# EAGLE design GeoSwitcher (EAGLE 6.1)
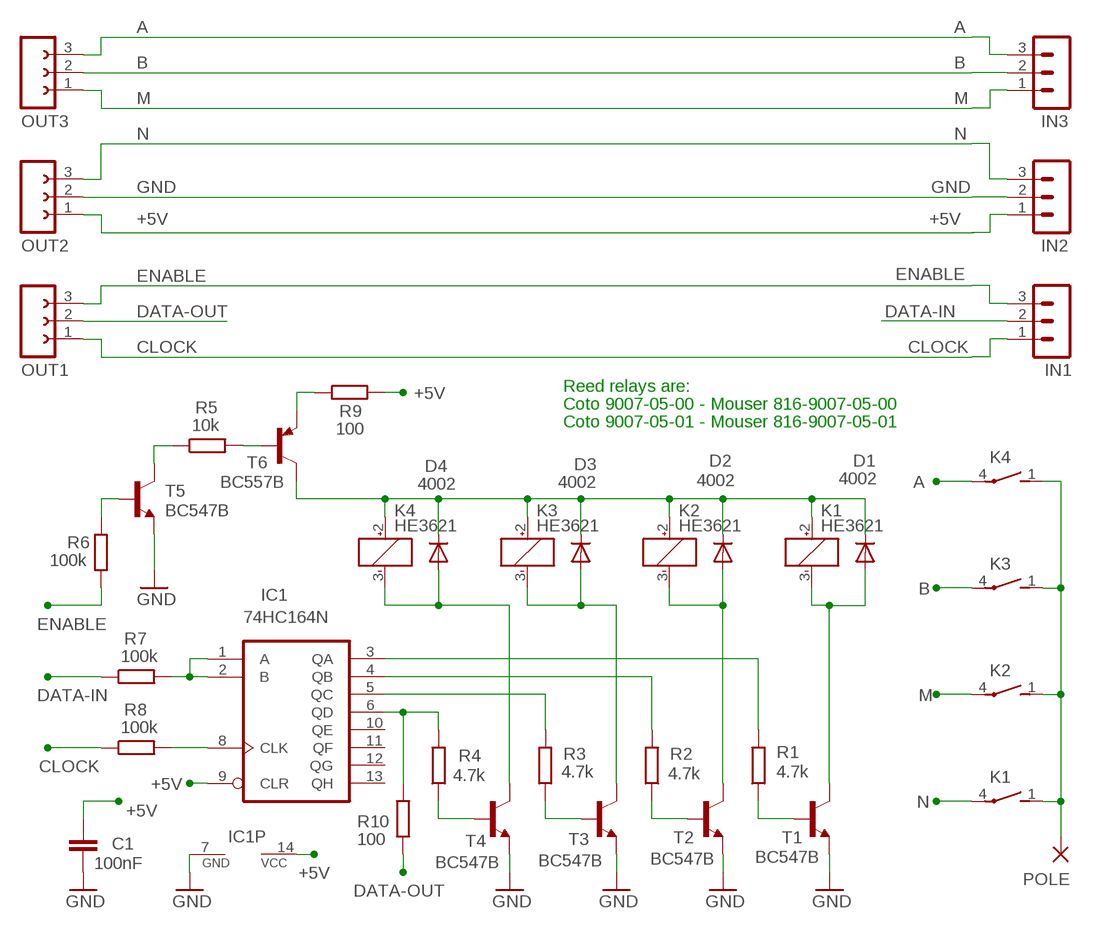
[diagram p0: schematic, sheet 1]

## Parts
C1  100nF  C-EU025-024X044  [C025-024X044]
D1  4002  DIODE-DO34-7  [DO34-7]
D2  4002  DIODE-DO34-7  [DO34-7]
D3  4002  DIODE-DO34-7  [DO34-7]
D4  4002  DIODE-DO34-7  [DO34-7]
IC1  74HC164N  [DIL14]
IN1  MA03-1N  [MA03-1]
IN2  MA03-1N  [MA03-1]
IN3  MA03-1N  [MA03-1]
K1  HE3621  [HE3621]
K2  HE3621  [HE3621]
K3  HE3621  [HE3621]
K4  HE3621  [HE3621]
OUT1  FE03-1"  [FE03-1]
OUT2  FE03-1"  [FE03-1]
OUT3  FE03-1"  [FE03-1]
POLE  WIREPAD2,54/0,8  [2,54/0,8]
R1  4.7k  R-EU_0204/7  [0204/7]
R2  4.7k  R-EU_0204/7  [0204/7]
R3  4.7k  R-EU_0204/7  [0204/7]
R4  4.7k  R-EU_0204/7  [0204/7]
R5  10k  R-EU_0204/7  [0204/7]
R6  100k  R-EU_0207/10  [0207/10]
R7  100k  R-EU_0207/12  [0207/12]
R8  100k  R-EU_0204/7  [0204/7]
R9  100  R-EU_0204/7  [0204/7]
R10  100  R-EU_0207/12  [0207/12]
T1  BC547B  -NPN-TO92-CBE  [TO92-CBE]
T2  BC547B  -NPN-TO92-CBE  [TO92-CBE]
T3  BC547B  -NPN-TO92-CBE  [TO92-CBE]
T4  BC547B  -NPN-TO92-CBE  [TO92-CBE]
T5  BC547B  -NPN-TO92-CBE  [TO92-CBE]
T6  BC557B  -PNP-TO92-CBE  [TO92-CBE]

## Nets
+5V: C1.1 IC1.9(CLR) IC1.14(VCC) IN2.1 OUT2.1 R9.2
A: IN3.3 K4.4(2:P) OUT3.3
B: IN3.2 K3.4(2:P) OUT3.2
CLOCK: IN1.1 OUT1.1 R8.1
DATA-IN: IN1.2 R7.1
DATA-OUT: OUT1.2 R10.1
ENABLE: IN1.3 OUT1.3 R6.2
GND: C1.2 IC1.7(GND) IN2.2 OUT2.2 T1.E T2.E T3.E T4.E T5.E
M: IN3.1 K2.4(2:P) OUT3.1
N: IN2.3 K1.4(2:P) OUT2.3
N$1: R4.1 T4.B
N$2: K1.1(2:S) K2.1(2:S) K3.1(2:S) K4.1(2:S) POLE.1(P)
N$3: D1.C D2.C D3.C D4.C K1.2(1:+) K2.2(1:+) K3.2(1:+) K4.2(1:+) T6.C
N$4: R3.1 T3.B
N$5: IC1.5(QC) R3.2
N$6: R2.1 T2.B
N$7: IC1.4(QB) R2.2
N$8: R1.1 T1.B
N$9: IC1.3(QA) R1.2
N$10: D4.A K4.3(1:-) T4.C
N$11: D3.A K3.3(1:-) T3.C
N$12: D2.A K2.3(1:-) T2.C
N$13: D1.A K1.3(1:-) T1.C
N$14: R5.1 T5.C
N$15: R5.2 T6.B
N$16: R6.1 T5.B
N$17: IC1.1(A) IC1.2(B) R7.2
N$18: IC1.8(CLK) R8.2
N$20: R9.1 T6.E
N$24: IC1.6(QD) R4.2 R10.2
Unconnected: IC1.10(QE) IC1.11(QF) IC1.12(QG) IC1.13(QH)

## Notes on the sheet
- Reed relays are:
- Coto 9007-05-00 - Mouser 816-9007-05-00
- Coto 9007-05-01 - Mouser 816-9007-05-01

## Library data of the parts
C1 = 00-LIVIO:C-EU: CAPACITOR, European symbol
D1-D4 = 00-LIVIO:DIODE-: DIODE
IC1 = 74xx-eu:74*164: 8-bit parallel out SHIFT REGISTER
IN1-IN3 = 03-con-lstb-M:MA03-1: PIN HEADER
K1-K4 = relay:HE3621: RELAY reed, 1 x norm. open, grid 5.08 mm, Hamlin
OUT1-OUT3 = 02-con-lsta-F:FE03-1: FEMALE HEADER
POLE = 00-LIVIO:WIREPAD: Wire PAD connect wire on PCB
R1-R10 = 00-LIVIO:R-EU_: RESISTOR, European symbol
T1-T5 = 00-LIVIO:*-NPN-: NPN Transistror
T6 = 00-LIVIO:*-PNP-: PNP Transistror

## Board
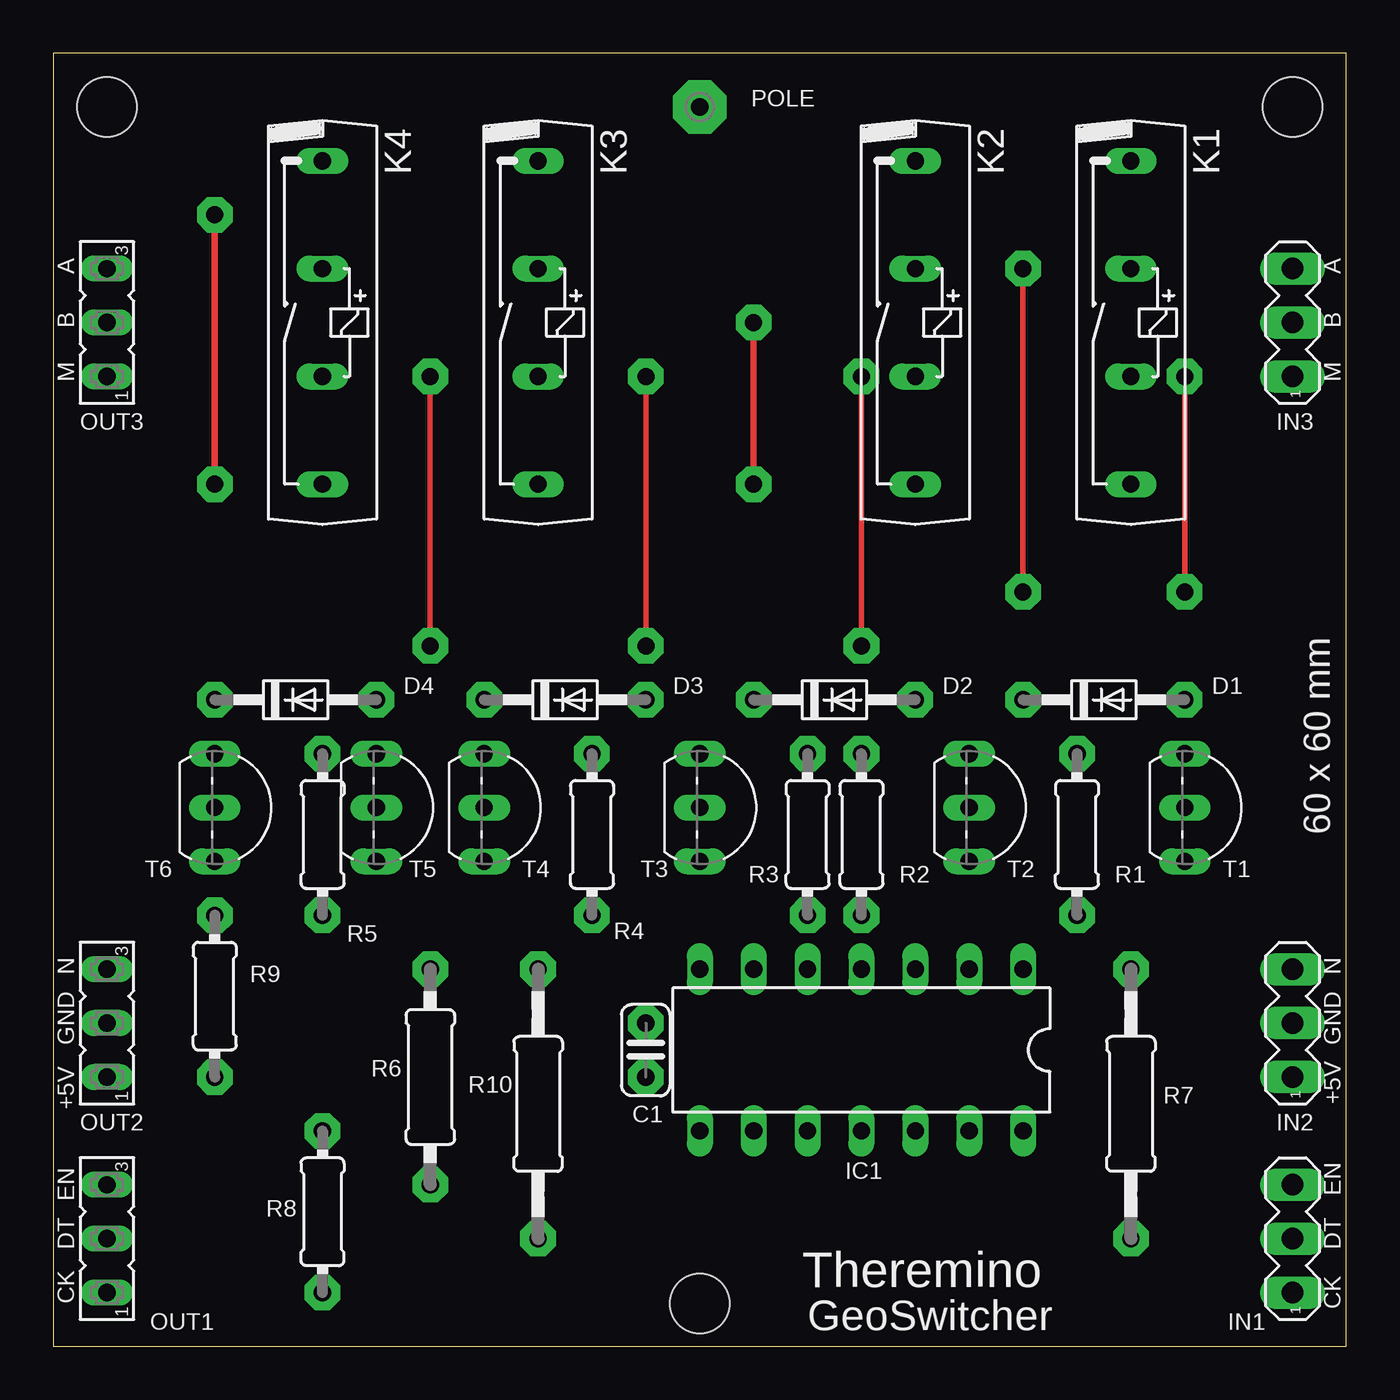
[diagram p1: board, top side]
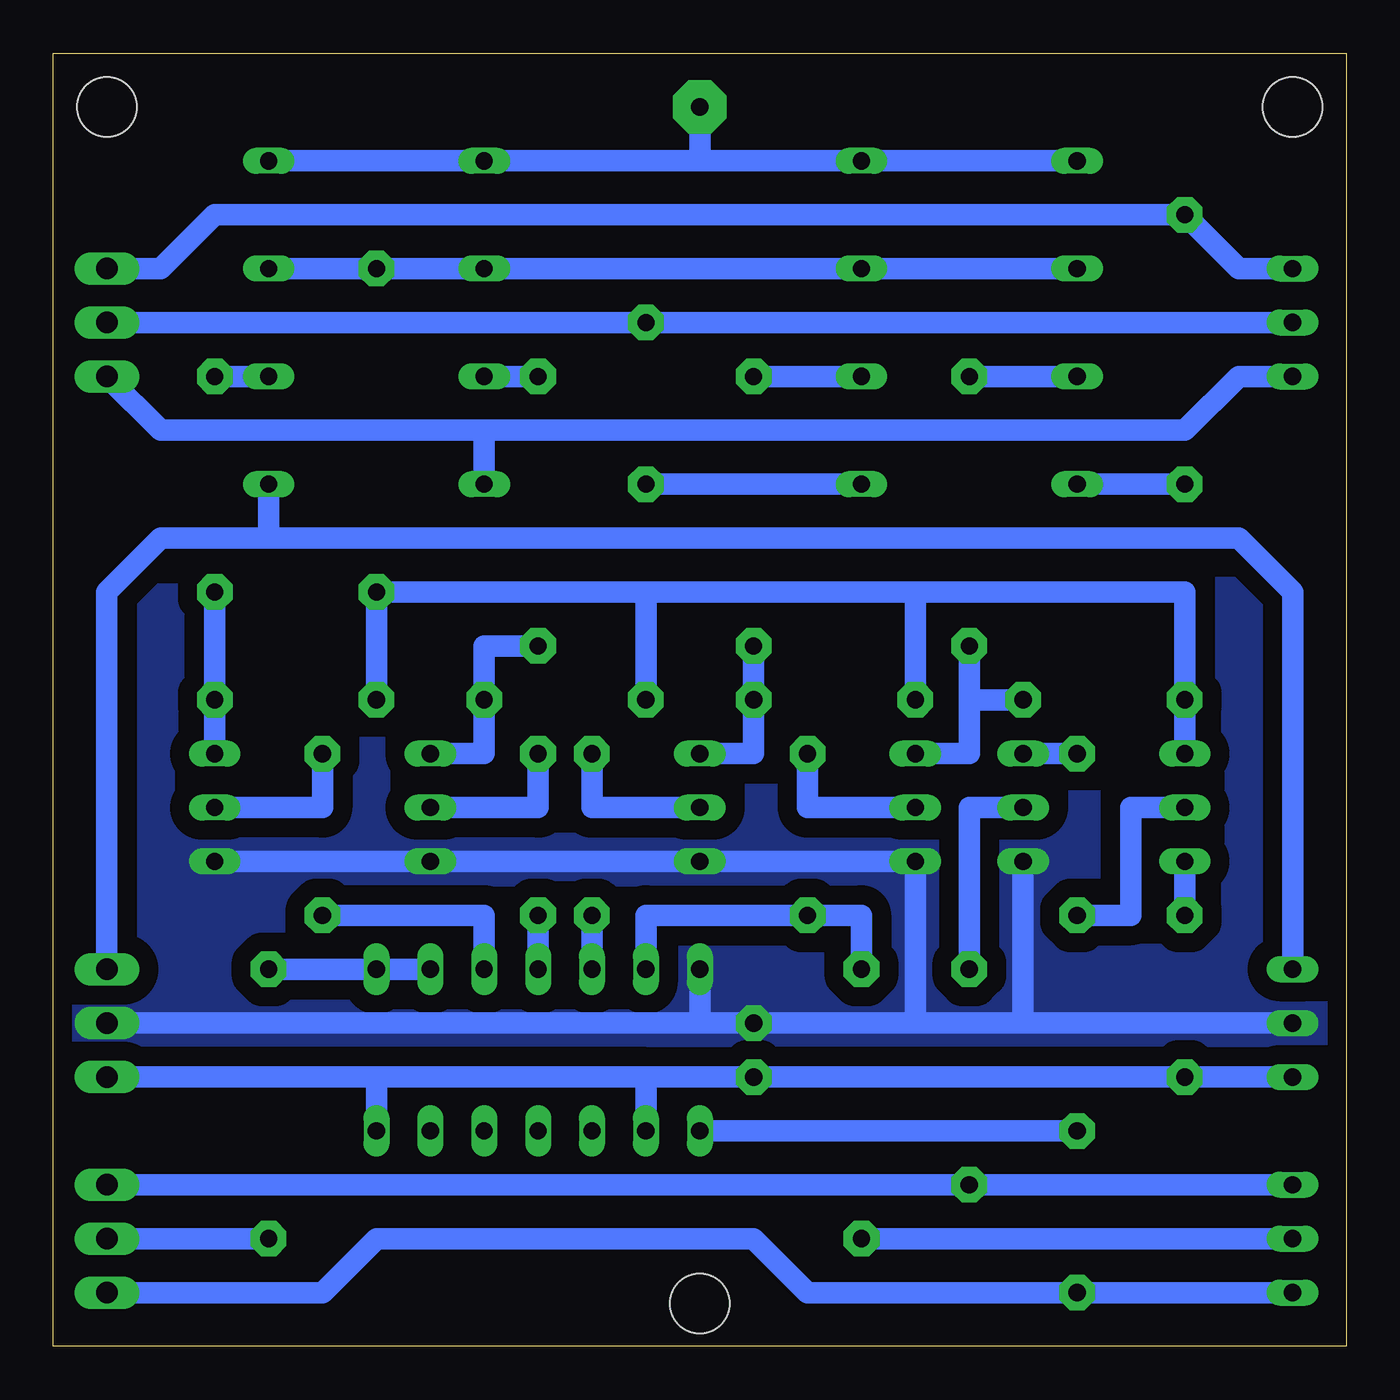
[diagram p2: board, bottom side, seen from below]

Size 60.96 x 60.96 mm. Coordinates in mm from the lower left corner, seen from the top.
Outline: 60.96,60.96 0,60.96 0,0 60.96,0 60.96,60.96
Copper layers (1*16): Top 0.035mm / dielectric 1.5mm / Bottom 0.035mm
Design rules: minimum track width 10mil, minimum drill 0.6mm, track to track 8mil, track to pad 8mil, pad to pad 8mil, via to via 8mil, smd to smd 8mil, copper to edge 31mil, drill to drill 8mil, minimum pad ring 5mil, minimum via ring 8mil, stop-mask expansion 4mil, vias tented up to drill 0mil, thermal gap 47mil
Holes 2.8 mm at 58.42,58.42 2.54,58.42 30.48,2.03

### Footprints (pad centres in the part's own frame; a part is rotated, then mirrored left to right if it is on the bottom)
C025-024X044 = drill 0.813 pad 1.676 octagon: 1 -1.27,0; 2 1.27,0
DO34-7 = drill 0.813 pad 1.676 octagon: A 3.81,0; C -3.81,0
DIL14 = drill 0.813 long: 1 -7.62,-3.81; 2 -5.08,-3.81; 3 -2.54,-3.81; 4 0,-3.81; 5 2.54,-3.81; 6 5.08,-3.81; 7 7.62,-3.81; 8 7.62,3.81; 9 5.08,3.81; 10 2.54,3.81; 11 0,3.81; 12 -2.54,3.81; 13 -5.08,3.81; 14 -7.62,3.81
MA03-1 = drill 1.016 long: 1 -2.54,0; 2 0,0; 3 2.54,0
HE3621 = drill 0.813 long: 1 -7.62,0; 2 -2.54,0; 3 2.54,0; 4 7.62,0
FE03-1 = drill 0.813 long: 1 -2.54,0; 2 0,0; 3 2.54,0
2,54/0,8 = drill 0.813 pad 2.54 octagon: 1 0,0
0204/7 = drill 0.813 pad 1.676 octagon: 1 -3.81,0; 2 3.81,0
0207/10 = drill 0.813 pad 1.676 octagon: 1 -5.08,0; 2 5.08,0
0207/12 = drill 0.813 pad 1.676 octagon: 1 -6.35,0; 2 6.35,0
TO92-CBE = drill 0.813 long: B 0,0; C -2.54,0; E 2.54,0

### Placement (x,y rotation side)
C1  27.94,13.97 90 top
D1  49.53,30.48 0 top
D2  36.83,30.48 0 top
D3  24.13,30.48 0 top
D4  11.43,30.48 0 top
IC1  38.1,13.97 180 top
IN1  58.42,5.08 90 top
IN2  58.42,15.24 90 top
IN3  58.42,48.26 90 top
K1  50.8,48.26 270 top
K2  40.64,48.26 270 top
K3  22.86,48.26 270 top
K4  12.7,48.26 270 top
OUT1  2.54,5.08 90 top
OUT2  2.54,15.24 90 top
OUT3  2.54,48.26 90 top
POLE  30.48,58.42 0 top
R1  48.26,24.13 270 top
R2  38.1,24.13 270 top
R3  35.56,24.13 270 top
R4  25.4,24.13 270 top
R5  12.7,24.13 270 top
R6  17.78,12.7 270 top
R7  50.8,11.43 90 top
R8  12.7,6.35 90 top
R9  7.62,16.51 270 top
R10  22.86,11.43 90 top
T1  53.34,25.4 270 top
T2  43.18,25.4 270 top
T3  30.48,25.4 270 top
T4  20.32,25.4 270 top
T5  15.24,25.4 270 top
T6  7.62,25.4 270 top

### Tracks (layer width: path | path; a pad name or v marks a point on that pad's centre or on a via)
+5V
  Bottom 1.016: IC1.9 33.02,12.7 | 33.02,12.7 45.72,12.7 | 45.72,12.7 IC1.14 | OUT2.1 R9.2 C1.1 33.02,12.7 | 45.72,12.7 IN2.1
A  (via drill 0.8 pad 1.68)
  Top 0.305: v7.62,40.64 v7.62,53.34
  Bottom 1.016: OUT3.3 5.08,50.8 v7.62,53.34 53.34,53.34 55.88,50.8 IN3.3 | K4.4 v7.62,40.64
B  (via drill 0.8 pad 1.68)
  Top 0.305: v33.02,40.64 v33.02,48.26
  Bottom 1.016: OUT3.2 5.08,48.26 v33.02,48.26 IN3.2 | K3.4 v33.02,40.64
CLOCK
  Bottom 1.016: OUT1.1 R8.1 25.4,2.54 27.94,5.08 45.72,5.08 48.26,2.54 IN1.1
DATA-IN
  Bottom 1.016: IN1.2 R7.1
DATA-OUT
  Bottom 1.016: OUT1.2 R10.1
ENABLE
  Bottom 1.016: IN1.3 R6.2 OUT1.3
GND
  Bottom 1.016: T1.E T2.E T3.E T4.E 20.32,15.24 | IC1.7 30.48,15.24 | 30.48,15.24 20.32,15.24 | 20.32,15.24 15.24,15.24 | 15.24,15.24 C1.2 OUT2.2 | 30.48,15.24 IN2.2 | T5.E 15.24,15.24
  pour Bottom (isolate 0.9, rank 6, no thermals): -1,-1 61.96,-1 61.96,61.96 -1,61.96
M
  Bottom 1.016: IN3.1 55.88,43.18 40.64,43.18 | 40.64,43.18 10.16,43.18 7.62,43.18 5.08,45.72 OUT3.1 | K2.4 40.64,43.18
N
  Bottom 1.016: 50.8,38.1 5.08,38.1 2.54,35.56 OUT2.3 | 50.8,38.1 55.88,38.1 58.42,35.56 IN2.3 | K1.4 50.8,38.1
N$1
  Bottom 1.016: R4.1 25.4,25.4 T4.B
N$2
  Bottom 1.016: K4.1 K3.1 30.48,55.88 | 30.48,55.88 K2.1 K1.1 | POLE.1 30.48,55.88
N$3  (via drill 0.8 pad 1.68)
  Top 0.254: v45.72,50.8 v45.72,35.56
  Bottom 1.016: T6.C D4.C 7.62,35.56 v45.72,35.56 | K1.2 K2.2 K3.2 K4.2 v45.72,50.8 | D3.C 20.32,35.56 | 20.32,35.56 v45.72,35.56 | D2.C 33.02,35.56 | 33.02,35.56 20.32,35.56 | D1.C v45.72,35.56 | v45.72,35.56 33.02,35.56
N$4
  Bottom 1.016: R3.1 35.56,25.4 T3.B
N$5
  Bottom 1.016: IC1.5 R3.2
N$6
  Bottom 1.016: R2.1 38.1,25.4 T2.B
N$7
  Bottom 1.016: IC1.4 R2.2
N$8
  Bottom 1.016: R1.1 48.26,25.4 T1.B
N$9
  Bottom 1.016: IC1.3 40.64,20.32 R1.2
N$10  (via drill 0.8 pad 1.68)
  Top 0.254: v17.78,33.02 v17.78,45.72
  Bottom 1.016: T4.C 17.78,27.94 17.78,30.48 | 17.78,30.48 D4.A 17.78,30.48 | 17.78,30.48 v17.78,33.02 | v17.78,45.72 K4.3
N$11  (via drill 0.8 pad 1.68)
  Top 0.254: v27.94,33.02 v27.94,45.72
  Bottom 1.016: T3.C 27.94,27.94 D3.A v27.94,33.02 | v27.94,45.72 K3.3
N$12  (via drill 0.8 pad 1.68)
  Top 0.254: v38.1,33.02 v38.1,45.72
  Bottom 1.016: T2.C 40.64,27.94 D2.A 40.64,33.02 v38.1,33.02 | v38.1,45.72 K2.3
N$13  (via drill 0.8 pad 1.68)
  Top 0.254: v53.34,35.56 v53.34,45.72
  Bottom 1.016: T1.C D1.A 53.34,32.38 v53.34,35.56 | v53.34,45.72 K1.3
N$14
  Bottom 1.016: T5.C R5.1
N$15
  Bottom 1.016: R5.2 10.16,20.32 10.16,25.4 T6.B
N$16
  Bottom 1.016: R6.1 17.78,25.4 T5.B
N$17
  Bottom 1.016: IC1.2 IC1.1 R7.2
N$18
  Bottom 1.016: IC1.8 R8.2
N$20
  Bottom 1.016: R9.1 T6.E
N$24
  Bottom 1.016: IC1.6 33.02,20.32 R4.2 22.86,20.32 R10.2

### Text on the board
tNames: A | A | B | B | M | M | 60 x 60 mm | N | N | GND | GND | +5V | +5V | EN | EN | DT | DT | Theremino | CK | CK | GeoSwitcher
